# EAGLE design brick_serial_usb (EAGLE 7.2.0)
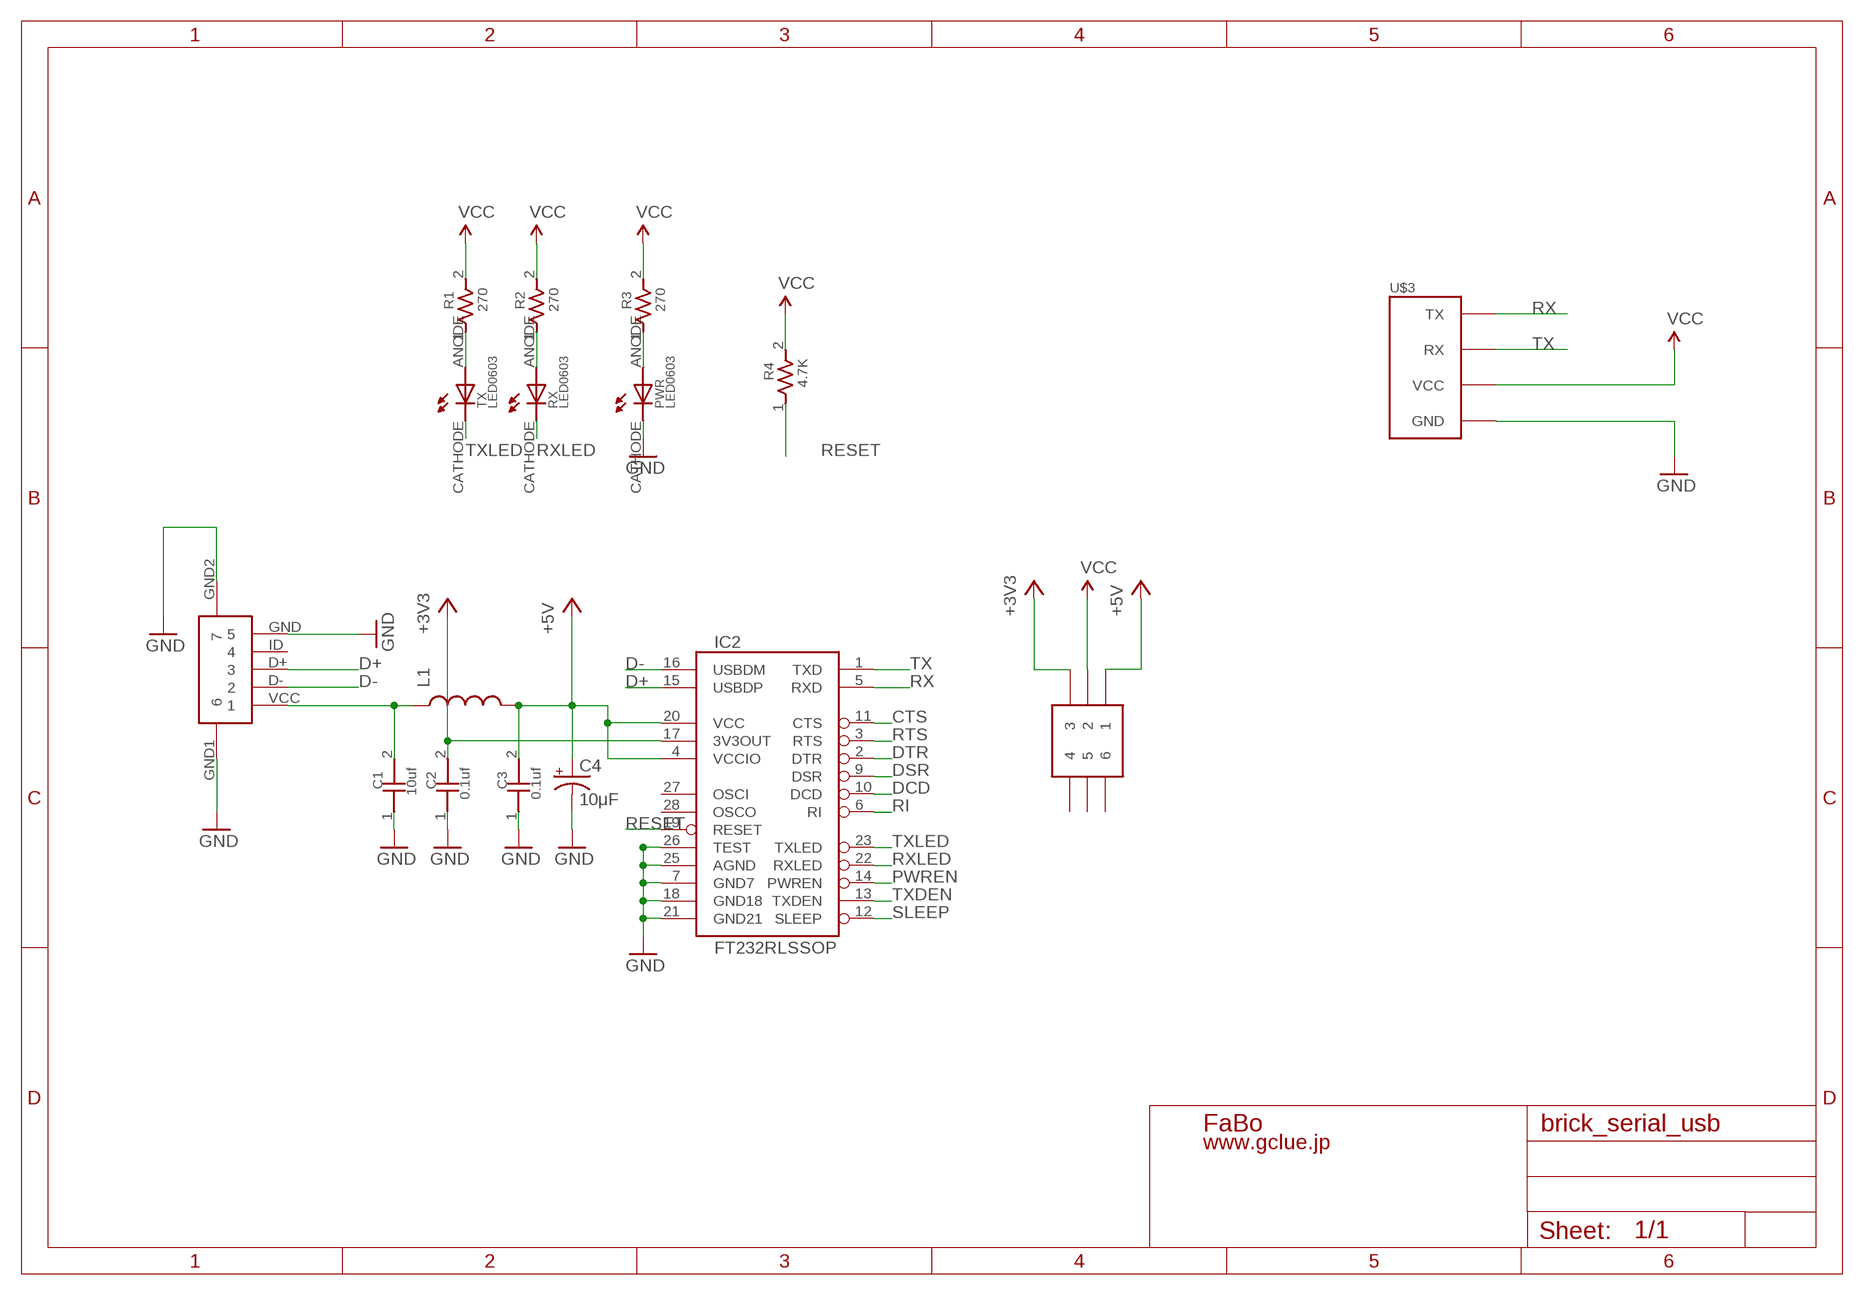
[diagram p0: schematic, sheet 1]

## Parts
C1  10uf  CAPACITOR0603  [0603]
C2  0.1uf  CAPACITOR0603  [0603]
C3  0.1uf  CAPACITOR0603  [0603]
C4  10μF  CAP_POL1206  [EIA3216]
IC2  FT232RLSSOP  [SSOP28DB]
L1  INDUCTOR0603  [0603]
PWR  LED0603  [0603]
R1  270  RESISTOR0603  [0603]
R2  270  RESISTOR0603  [0603]
R3  270  RESISTOR0603  [0603]
R4  4.7K  RESISTOR0603  [0603]
RX  LED0603  [0603]
TX  LED0603  [0603]
U$1  USB-MICRO-B-FEMALE  [USB-MICRO-B-FEMALE]
U$2  C&K_JS202011SCQN  [C&K_JS202011SCQN]
U$3  BRICK_SERIAL  [BRICK_SERIAL]

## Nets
+3V3: C2.2 IC2.17(3V3OUT) U$2.3
+5V: C3.2 C4.A(+) IC2.4(VCCIO) IC2.20(VCC) L1.2 U$2.1
CTS: IC2.11(CTS)
D+: IC2.15(USBDP) U$1.D+
D-: IC2.16(USBDM) U$1.D-
DCD: IC2.10(DCD)
DSR: IC2.9(DSR)
DTR: IC2.2(DTR)
GND: C1.1 C2.1 C3.1 C4.C(-) IC2.7(GND7) IC2.18(GND18) IC2.21(GND21) IC2.25(AGND) IC2.26(TEST) PWR.CATHODE U$1.GND U$1.GND1 U$1.GND2 U$3.GND
N$1: C1.2 L1.1 U$1.VCC
N$2: R1.1 TX.ANODE
N$5: R2.1 RX.ANODE
N$6: PWR.ANODE R3.1
PWREN: IC2.14(PWREN)
RESET: IC2.19(RESET) R4.1
RI: IC2.6(RI)
RTS: IC2.3(RTS)
RX: IC2.5(RXD) U$3.TX
RXLED: IC2.22(RXLED) RX.CATHODE
SLEEP: IC2.12(SLEEP)
TX: IC2.1(TXD) U$3.RX
TXDEN: IC2.13(TXDEN)
TXLED: IC2.23(TXLED) TX.CATHODE
VCC: R1.2 R2.2 R3.2 R4.2 U$2.2 U$3.VCC
Unconnected: IC2.27(OSCI) IC2.28(OSCO) U$1.ID U$2.4 U$2.5 U$2.6

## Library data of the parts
C1-C3 = GClue-Capacitor:CAPACITOR
C4 = SparkFun:CAP_POL: Capacitor Polarized
IC2 = SparkFun:FT232RL: USB UART FT232RL 4th Generation USB UART (USB <-> Serial) Controller. Spark Fun Electronics SKU : COM-00650
L1 = SparkFun:INDUCTOR: Inductors
PWR RX TX = GClue-LED:LED
R1-R4 = GClue-Resistors:RESISTOR
U$1 = gclue:USB-MICRO-B-FEMALE
U$2 = gclueParts:C&K_JS202011SCQN
U$3 = gclue:BRICK_SERIAL: FaBo Brick 4pin(SERIAL)

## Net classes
0 default: width 0.254 mm

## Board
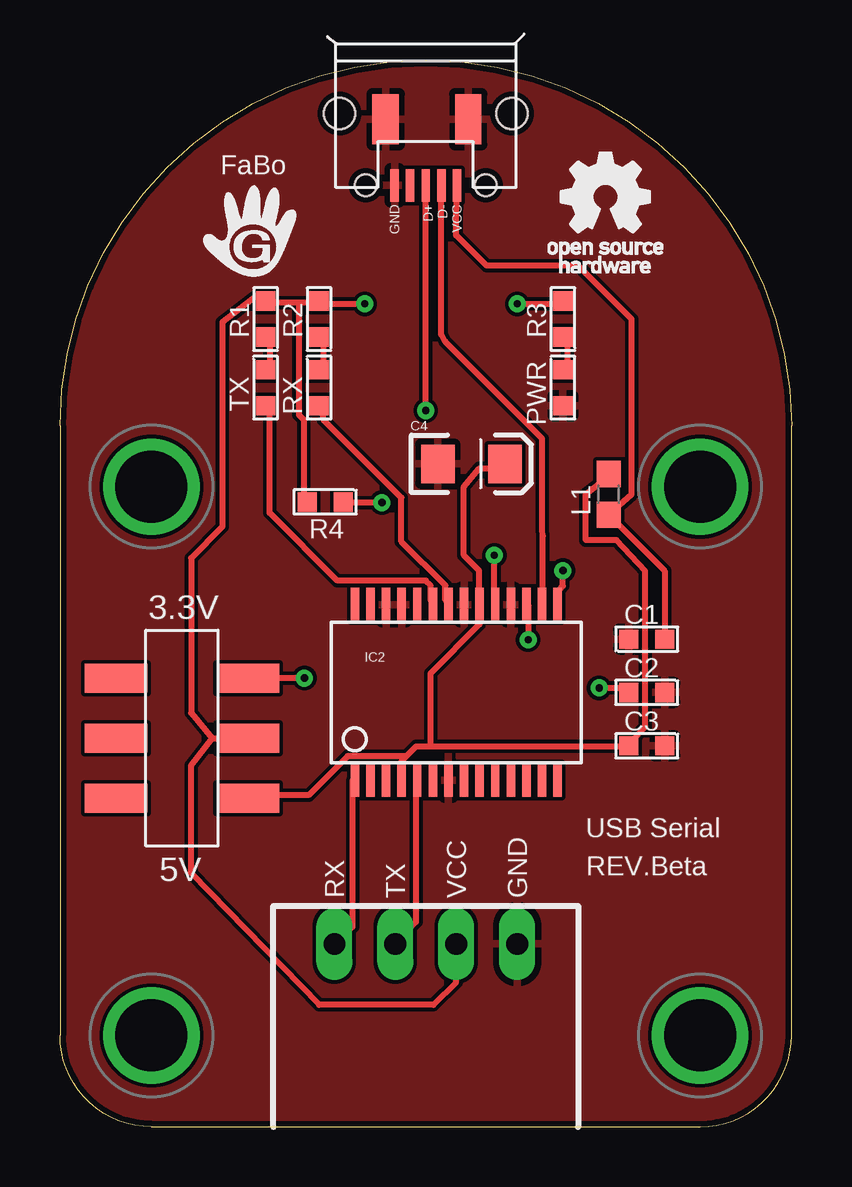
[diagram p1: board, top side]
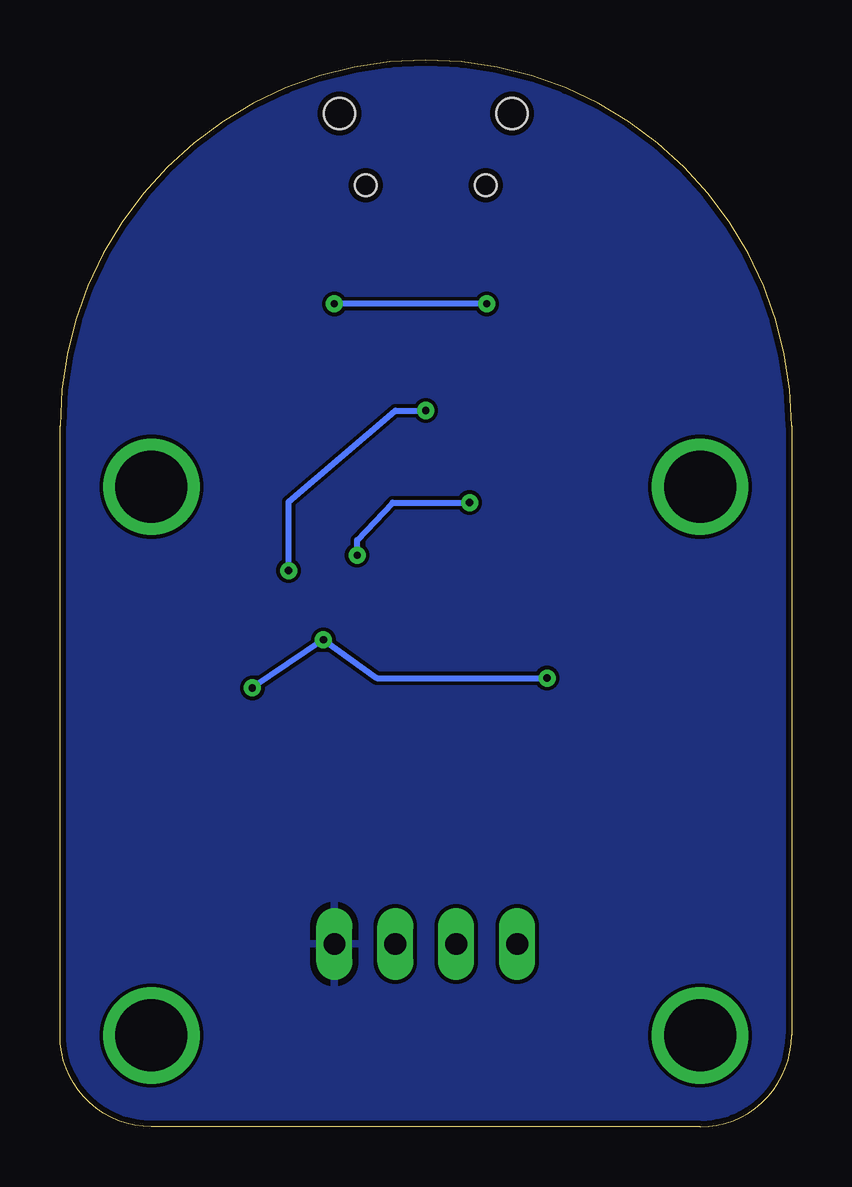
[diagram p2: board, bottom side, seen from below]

Size 30.48 x 44.45 mm. Coordinates in mm from the lower left corner, seen from the top.
Copper layers (1*16): Top 0.035mm / dielectric 1.5mm / Bottom 0.035mm
Design rules "DFRobot_Eagle_Rule_v0.4": minimum track width 6mil, minimum drill 12mil, track to track 6mil, track to pad 6mil, pad to pad 6mil, via to via 6mil, smd to smd 0mil, copper to edge 10mil, drill to drill 10mil, minimum pad ring 12mil, minimum via ring 8mil, stop-mask expansion 2mil, vias tented up to drill 25mil, thermal gap 10mil

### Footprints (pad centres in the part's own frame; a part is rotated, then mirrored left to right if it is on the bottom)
0603 = smd 0.8 x 0.8: 1 -0.75,0; 2 0.75,0
EIA3216 = smd 1.4 x 1.6: A 1.4,0; C -1.4,0
SSOP28DB = smd 0.348 x 1.397: 1 -4.225,-3.656; 2 -3.575,-3.656; 3 -2.925,-3.656; 4 -2.275,-3.656; 5 -1.625,-3.656; 6 -0.975,-3.656; 7 -0.325,-3.656; 8 0.325,-3.656; 9 0.975,-3.656; 10 1.625,-3.656; 11 2.275,-3.656; 12 2.925,-3.656; 13 3.575,-3.656; 14 4.225,-3.656; 15 4.225,3.656; 16 3.575,3.656; 17 2.925,3.656; 18 2.275,3.656; 19 1.625,3.656; 20 0.975,3.656; 21 0.325,3.656; 22 -0.325,3.656; 23 -0.975,3.656; 24 -1.625,3.656; 25 -2.275,3.656; 26 -2.925,3.656; 27 -3.575,3.656; 28 -4.225,3.656
0603' = smd 1.1 x 1: 1 -0.85,0; 2 0.85,0
0603'' = smd 0.8 x 0.8: ANODE -0.75,0; CATHODE 0.75,0
USB-MICRO-B-FEMALE = smd 1.35 x 0.35: D+ 3,0; D- 3,0.65; GND 3,-1.3; ID 3,-0.65; VCC 3,1.3 | smd 2.1 x 1.1: GND1 0.246,1.77; GND2 0.246,-1.67 | hole 1.3: 0,3.6; 0,-3.6 | hole 0.9: 3,2.5; 3,-2.5
C&K_JS202011SCQN = smd 2.6 x 1.2: 1 -2.75,2.5; 2 -2.75,0; 3 -2.75,-2.5; 4 2.75,-2.5; 5 2.75,0; 6 2.75,2.5
BRICK_SERIAL = drill 0.9 long: GND 3.81,-11.43; RX -3.81,-11.43; TX -1.27,-11.43; VCC 1.27,-11.43 | drill 3 pad 3.81: P$5 -11.43,7.62; P$6 11.43,7.62; P$7 -11.43,-15.24; P$8 11.43,-15.24

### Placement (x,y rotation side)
C1  24.45,20.32 0 top
C2  24.45,18.1 180 top
C3  24.45,15.88 180 top
C4  17.14,27.62 0 top
IC2  16.51,18.1 0 top
L1  [0603']  22.86,26.35 90 top
PWR  LED0603  [0603'']  20.95,30.8 270 top
R1  8.57,33.66 90 top
R2  10.79,33.66 90 top
R3  20.95,33.66 90 top
R4  11.05,26.04 180 top
RX  LED0603  [0603'']  10.79,30.8 270 top
TX  LED0603  [0603'']  8.57,30.8 270 top
U$1  15.24,42.23 270 top
U$2  5.08,16.19 180 top
U$3  15.24,19.05 0 top
U$5  [LOGO_GCLUE_M]  7.87,37.34 0 top
U$6  [LOGO_OSHW_T_M]  22.86,38.1 0 top

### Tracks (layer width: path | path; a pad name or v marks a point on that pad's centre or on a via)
+3V3  (via drill 0.3)
  Top 0.254: v22.47,18.29 23.57,18.29 C2.2 | v19.51,20.3 19.51,21.74 IC2.17 | v10.19,18.69 7.92,18.69 U$2.3
  Bottom 0.254: v22.47,18.29 v19.51,20.3 17.27,18.69 v10.19,18.69
+5V
  Top 0.254: 15.44,15.85 14.83,15.85 14.43,15.44 | 15.44,15.85 23.57,15.85 C3.2 23.77,16.05 24.38,16.66 24.38,23.15 23.18,24.45 21.91,24.45 21.91,26.35 22.76,27.03 L1.2 | 14.43,15.44 14.22,15.24 14.22,14.63 IC2.4 | 15.44,15.85 15.44,18.9 17.48,20.93 17.48,21.74 IC2.20 17.48,21.95 17.46,22.23 17.46,23.18 16.83,23.81 16.83,26.67 17.48,27.43 18.49,27.43 C4.A | 14.43,15.44 11.99,15.44 10.36,13.82 7.92,13.82 U$2.1
D+  (via drill 0.3)
  Top 0.254: v15.24,29.84 U$1.D+ | v20.95,23.18 20.95,22.54 20.73,22.26 IC2.15
  Bottom 0.254: v20.95,23.18 20.95,26.04 16.51,29.84 v15.24,29.84
D-
  Top 0.254: U$1.D- 15.88,33.02 16.05,32.72 20.09,28.68 20.09,24.91 20.12,24.61 20.12,21.95 IC2.16
GND
  pour Bottom: -0.64,-0.64 31.11,-0.64 31.11,46.35 -0.64,46.35
  pour Top: -0.64,-0.64 31.11,-0.64 31.11,46.35 -0.64,46.35
N$1
  Top 0.254: C1.2 25.2,23.16 22.96,25.4 L1.1 22.96,25.6 23.81,26.35 23.81,33.66 21.59,35.88 17.78,35.88 16.51,37.15 U$1.VCC
N$2
  Top 0.254: TX.ANODE 8.74,31.7 8.74,32.72 R1.1
N$5
  Top 0.254: RX.ANODE 10.97,31.7 10.97,32.72 R2.1
N$6
  Top 0.254: PWR.ANODE 21.13,31.7 21.13,32.72 R3.1
RESET  (via drill 0.3)
  Top 0.254: v13.41,26.01 11.99,26.01 R4.1 | v18.1,23.81 18.1,21.91 IC2.19
  Bottom 0.254: v13.41,26.01 16.62,26.01 18.1,24.45 v18.1,23.81
RX
  Top 0.254: IC2.5 14.83,14.43 14.83,8.53 14.02,7.72 U$3.TX
RXLED
  Top 0.254: RX.CATHODE 10.97,29.87 10.97,29.46 14.22,26.21 14.22,24.38 16.05,22.55 16.05,21.95 IC2.22
TX
  Top 0.254: IC2.1 12.19,14.43 12.19,8.33 11.58,7.72 U$3.RX
TXLED
  Top 0.254: TX.CATHODE 8.74,29.87 8.74,25.58 11.56,22.76 15.24,22.76 15.44,22.55 15.44,21.95 IC2.23
VCC  (via drill 0.3)
  Top 0.254: 6.35,16.19 5.46,15.06 5.46,10.57 10.79,5.08 15.56,5.08 16.51,6.03 U$3.VCC | 6.35,16.19 7.72,16.05 U$2.2 7.72,16.26 6.35,16.19 | 9.96,34.34 10.77,34.34 R2.2 10.79,34.29 v12.7,34.29 | 9.96,34.34 8.74,34.34 R1.2 8.22,34.66 6.77,33.53 6.77,25.01 5.46,23.7 5.46,17.25 6.35,16.19 | 9.96,34.34 9.96,29.67 10.16,29.46 10.16,26.21 R4.2 | v19.05,34.29 20.95,34.29 R3.2
  Bottom 0.254: v12.7,34.29 v19.05,34.29

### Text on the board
tPlace: FaBo | 3.3V | USB Serial | 5V | REV.Beta

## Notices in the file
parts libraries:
SparkFun: Licensing: CC v3.0 Share-Alike You are welcome to use this library for commercial purposes.
